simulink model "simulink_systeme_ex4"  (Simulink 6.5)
settings: Solver=ode3  StartTime=0.0  StopTime=.5  FixedStep=0.001  RelTol=1e-3
PostLoadFcn:
  | simulink_systems_ex1
  | simulink_systems_ex2
  | simulink_systems_ex3
  | simulink_systems_ex4
InitFcn:
  | simulink_systems_ex1
  | simulink_systems_ex2
  | simulink_systems_ex3
  | simulink_systems_ex4
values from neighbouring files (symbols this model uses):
  A = [-2*D*w -w^2 ; 1 0]    [simulink_systems_ex3.m]
  B = [w^2 ; 0 ]    [simulink_systems_ex3.m]
  C = [0 1]    [simulink_systems_ex3.m]
  D = 0    [simulink_systems_ex3.m]
  T1 = 0.01    [simulink_systems_ex1.m]
  Ti = 0.1    [simulink_systems_ex2.m]
  Tm = 0.001    [simulink_systems_ex4.m]
  V = 1    [simulink_systems_ex1.m]
  Vm = 1    [simulink_systems_ex4.m]

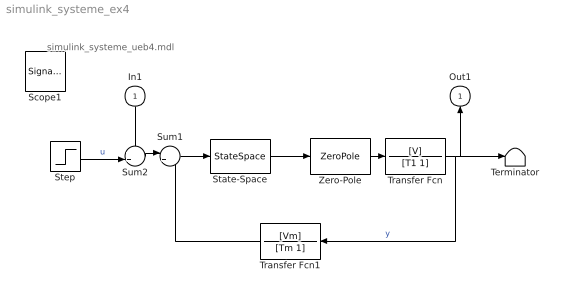
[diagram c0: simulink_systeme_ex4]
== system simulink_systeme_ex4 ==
  note: simulink_systeme_ueb4.mdl
  In1 : Inport  Orientation=down
  State-Space : StateSpace  A=A  B=B  C=C  D=D
  Step : Step  Time=.1  SampleTime=0
  Sum1 : Sum  Inputs=|+-
  Sum2 : Sum  Inputs=++|
  Terminator : Terminator
  Transfer Fcn : TransferFcn  Numerator=[V]  Denominator=[T1 1]
  Transfer Fcn1 : TransferFcn  Orientation=left  Numerator=[Vm]  Denominator=[Tm 1]
  Zero-Pole : ZeroPole  Zeros=[]  Poles=[0]  Gain=1/Ti
  Out1 : Outport  Orientation=up
  Scope1 : SignalViewerScope  IOType=viewer  NumInputPorts=4  RefreshTime=0.035000
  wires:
  State-Space/1 -> Zero-Pole/1
  Zero-Pole/1 -> Transfer Fcn/1
  Sum1/1 -> State-Space/1
  Transfer Fcn/1 -> Transfer Fcn1/1, Terminator/1, Out1/1  "y"
  Step/1 -> Sum2/2  "u"
  Transfer Fcn1/1 -> Sum1/2
  In1/1 -> Sum2/1
  Sum2/1 -> Sum1/1
